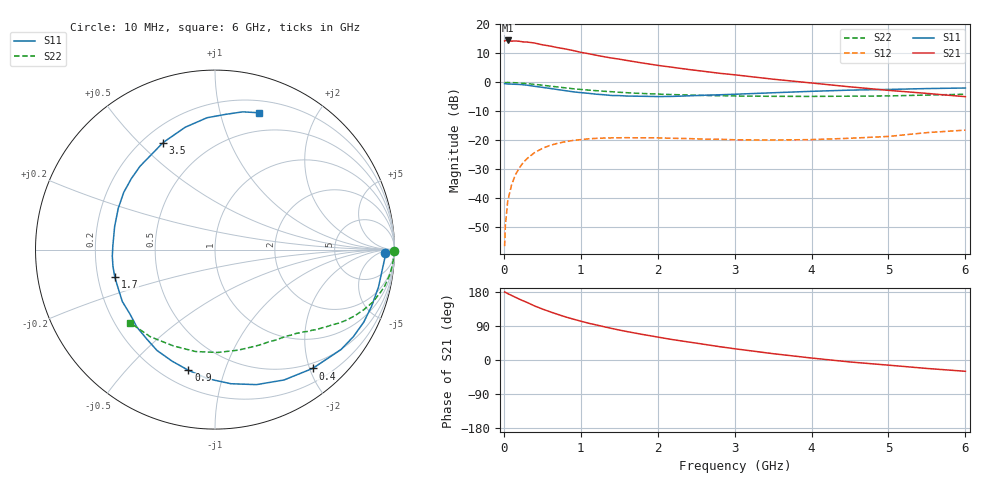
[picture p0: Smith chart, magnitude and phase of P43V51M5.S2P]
! SIEMENS Small Signal Semiconductors
! BFP182
! Si NPN RF Bipolar Junction Transistor in SOT143
! VCE = 3.5 V  IC = 1.5 mA
! Common Emitter S-Parameters:  March  1996
# GHz  S  MA  R  50
!  f  S11  S21  S12  S22
! GHz  MAG  ANG  MAG  ANG  MAG  ANG  MAG  ANG
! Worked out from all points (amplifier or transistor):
!   36 points, 10 MHz to 6 GHz, reference 50 ohm
!   highest |S21| = 14.5 dB at 50 MHz (marker M1)
!   |S21| within 3 dB of that: start of sweep to 813.8 MHz
!   unconditionally stable (mu >= 1): 2.415 GHz to end of sweep
!   at 250 MHz: K = 0.11, MSG = 20.8 dB, |S12| = -27.7 dB
!   at 1.4 GHz: K = 0.60, MSG = 13.8 dB, |S12| = -19.1 dB
!   at 6 GHz: K = 1.02, MAG = 4.9 dB, |S12| = -16.4 dB
!   S11 on the Smith chart (normalised r, x): 10 MHz: 33, -13; 400 MHz: 0.41, -2.05; 900 MHz: 0.30, -0.76; 1.7 GHz: 0.27, -0.13; 3.5 GHz: 0.28, +0.59; 6 GHz: 0.31, +1.32
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0.01  0.9483 -1.2  5.184 179.3  0.0015 85.4  0.9983 -0.4
0.02  0.948 -2.6  5.274 178.7  0.0034 92.1  0.9919 -1.0
0.05  0.9392 -6.5  5.286 175.2  0.0089 87.1  0.9969 -2.4
0.1  0.9345 -12.9  5.148 170.4  0.017 81.2  0.9917 -4.9
0.15  0.9279 -19.8  5.188 165.6  0.0255 78.1  0.9864 -7.5
0.2  0.9221 -26.0  5.122 160.8  0.0333 74.7  0.9765 -9.8
0.25  0.9108 -32.2  4.991 156.2  0.0412 70.9  0.9672 -12.1
0.3  0.8962 -38.4  4.968 152.1  0.0484 66.6  0.9535 -14.3
0.4  0.8568 -50.6  4.771 142.6  0.0616 60.4  0.9258 -18.5
0.5  0.8219 -62.1  4.453 134.6  0.0727 53.7  0.8941 -22.0
0.6  0.7871 -72.9  4.236 127.3  0.0821 48.3  0.8631 -25.2
0.8  0.7206 -93.2  3.775 113.8  0.0949 38.6  0.8051 -30.5
0.9  0.6885 -102.4  3.543 108.0  0.0998 34.8  0.7773 -32.6
1.1  0.6483 -119.9  3.13 97.1  0.1062 27.9  0.7363 -36.4
1.4  0.5943 -142.9  2.634 83.4  0.1105 19.9  0.6907 -41.3
1.7  0.579 -164.6  2.272 71.3  0.1107 14.8  0.6517 -45.7
2.2  0.5738 167.0  1.815 53.6  0.1086 9.2  0.616 -53.0
2.8  0.6113 139.7  1.438 35.3  0.1045 6.7  0.5898 -63.0
3.5  0.6627 115.9  1.136 16.7  0.1014 8.3  0.575 -76.9
4.5  0.7359 93.5  0.838 -5.2  0.1088 13.8  0.5782 -100.8
5.5  0.7829 78.6  0.646 -22.3  0.1361 17.5  0.6047 -126.6
6  0.8004 72.3  0.567 -29.8  0.1505 15.1  0.6247 -139.3
